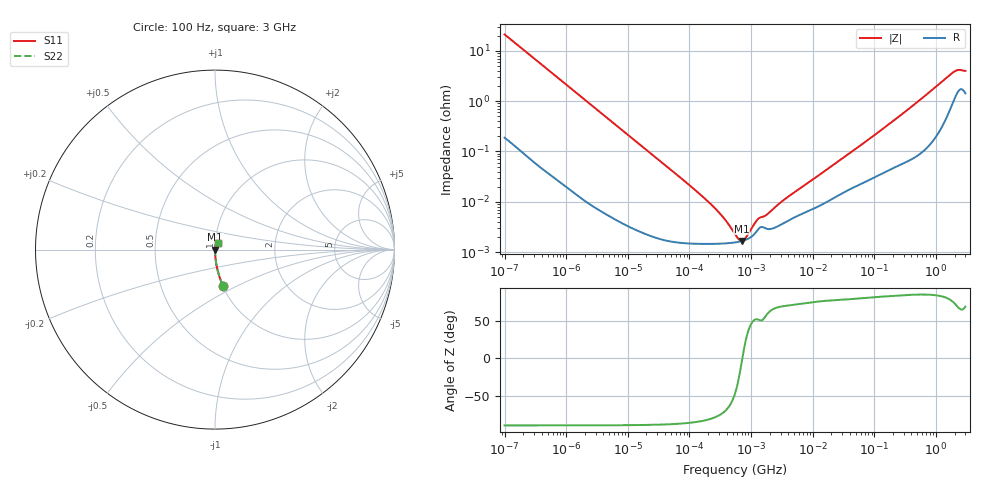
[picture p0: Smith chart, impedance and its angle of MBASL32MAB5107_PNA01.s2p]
! MBASL32MAB5107_PNA01  S-PARAMETER MODEL  ( Standard Model )
! Model Generated by TAIYO YUDEN Corporation (http://www.ty-top.com)
! Version 1.0
! TAIYO YUDEN Control No. 220601
! Copyright(c) 2015 TAIYO YUDEN CO.,LTD. All Rights Reserved.
! Product Description (link to TY-COMPAS)
! https://ds.yuden.co.jp/TYCOMPAS/or/detail?pn=MBASL32MAB5107MPNA01&u=M
! Products Name : Multilayer Ceramic Capacitors
! Characteristics :
!  Capacitance : 100 [uF] , Rated Voltage : 10 [V] , TCC : X5R
!  Case Size : 3.2 x 2.5 / 0.126 x 0.098 [mm/inch] , Thickness : 2.5 / 0.098 [mm/inch]
!  (Conditions: Temperature = 25 [degC] , DC Bias Voltage = 0 [V])
! External Node Assignments :
!  1  o---| |---o  2
! GND o---------o GND
! Frequency Range : 100Hz  -  3GHz  [ 401 STEP ]
# MHZ S RI R 50
! Freq[MHz].  S11 Real  S11 Imag  S21 Real  S21 Imag  S12 Real  S12 Imag  S22 Real  S22 Imag
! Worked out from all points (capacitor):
!   401 points, 100 Hz to 3 GHz, reference 50 ohm
!   read as one part in series: C = 75.6 uF near 109 Hz
!   lowest |Z| = 1.67 mohm at 709.1 kHz (marker M1)
!   series resonance near 720.3 kHz, so ESL is about 650 pH
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0.0001  0.0439 -0.2005  0.9561 0.2005  0.9561 0.2005  0.0439 -0.2005
0.000114  0.0345 -0.1782  0.9655 0.1782  0.9655 0.1782  0.0345 -0.1782
0.000175  0.0153 -0.1185  0.9847 0.1185  0.9847 0.1185  0.0153 -0.1185
0.000348  0.0042 -0.0605  0.9958 0.0605  0.9958 0.0605  0.0042 -0.0605
0.000724  0.00113 -0.0293  0.9989 0.0293  0.9989 0.0293  0.00113 -0.0293
0.001788  0.000258 -0.0119  0.9997 0.0119  0.9997 0.0119  0.000258 -0.0119
0.031977  1.9e-05 -0.000678  1 0.000678  1 0.000678  1.9e-05 -0.000678
0.089839  1.51e-05 -0.000239  1 0.000239  1 0.000239  1.51e-05 -0.000239
0.194955  1.46e-05 -0.000104  1 0.000104  1 0.000104  1.46e-05 -0.000104
0.221826  1.47e-05 -8.9e-05  1 8.9e-05  1 8.9e-05  1.47e-05 -8.9e-05
0.547723  1.57e-05 -1.69e-05  1 1.69e-05  1 1.69e-05  1.57e-05 -1.69e-05
0.709116  1.67e-05 -9.47e-07  1 9.47e-07  1 9.47e-07  1.67e-05 -9.47e-07
2.81117  3.35e-05 8.46e-05  1 -8.46e-05  1 -8.46e-05  3.35e-05 8.46e-05
3.063887  3.54e-05 9.26e-05  1 -9.26e-05  1 -9.26e-05  3.54e-05 9.26e-05
9.794414  7.13e-05 0.000263  0.9999 -0.000263  0.9999 -0.000263  7.13e-05 0.000263
54.78865  0.000215 0.00121  0.9998 -0.00121  0.9998 -0.00121  0.000215 0.00121
175.1444  0.000442 0.00351  0.9996 -0.00351  0.9996 -0.00351  0.000442 0.00351
492.0662  0.000901 0.00943  0.9991 -0.00943  0.9991 -0.00943  0.000901 0.00943
1868.531  0.0103 0.0349  0.9897 -0.0349  0.9897 -0.0349  0.0103 0.0349
2126.076  0.0144 0.0372  0.9856 -0.0372  0.9856 -0.0372  0.0144 0.0372
2317.205  0.017 0.0373  0.983 -0.0373  0.983 -0.0373  0.017 0.0373
3000  0.0153 0.0361  0.9847 -0.0361  0.9847 -0.0361  0.0153 0.0361
